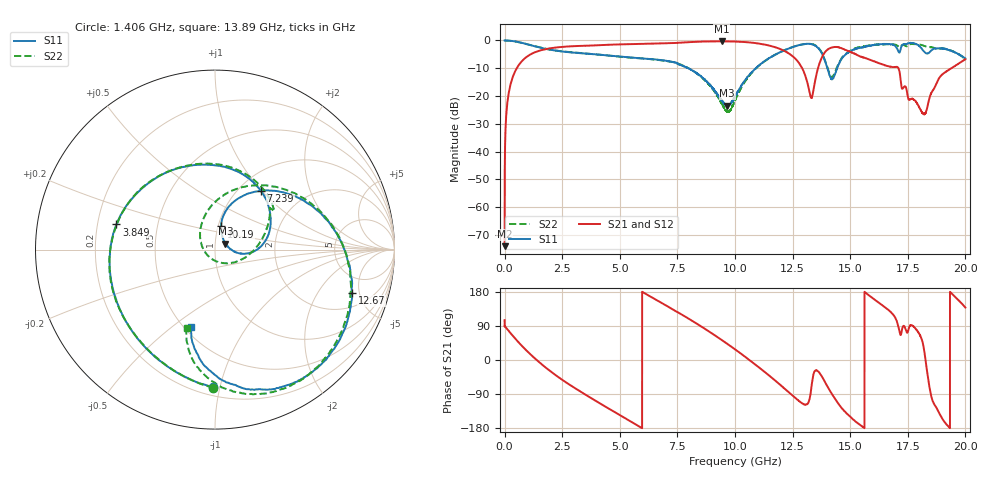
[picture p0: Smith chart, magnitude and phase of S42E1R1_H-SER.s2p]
! Created Wed Nov 25 21:31:11 2020
# khz S ma R 50
! 2 Port Network Data from SP1.SP block
! freq  magS11  angS11  magS21  angS21  magS12  angS12  magS22  angS22
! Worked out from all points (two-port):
!   20001 points, 300 kHz to 20 GHz, reference 50 ohm
!   highest |S21| = -0.32 dB at 9.429 GHz (marker M1); lowest = -74.1 dB at 300 kHz (marker M2)
!   |S21| within 3 dB of the highest: 1.675 GHz to 12.03 GHz (10.35 GHz wide, 151 % of centre); 14.01 GHz to 14.77 GHz (753.6 MHz wide, 5.24 % of centre)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
!   lowest |S11| = -23.5 dB at 9.663 GHz (marker M3), VSWR 1.14, Z = 56 + j3.78 ohm
!   |S11| at or under -10 dB: 7.968565 GHz to 7.970692 GHz (2.127 MHz wide, 0.0267 % of centre); 7.972 GHz to 10.9 GHz (2.929 GHz wide, 31 % of centre); 14.01 GHz to 14.44 GHz (424.7 MHz wide, 2.99 % of centre)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
!   |S22| runs from -25.8 to 0.0 dB; largest |S21 - S12| = 0.012
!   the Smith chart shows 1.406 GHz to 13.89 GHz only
!   S11 on the Smith chart (normalised r, x): 1.406 GHz: 0.26, -0.95; 3.849 GHz: 0.28, +0.12; 7.239 GHz: 1.26, +0.99; 10.19 GHz: 1.03, +0.27; 12.67 GHz: 3.16, -4.21; 13.89 GHz: 0.55, -0.58
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300  0.9984 -0.2  0.0001982 105.2  0.0002223 95.0  0.9986 -0.3
107300  0.9968 -7.9  0.06836 81.9  0.06863 82.0  0.9976 -7.8
255300  0.9847 -18.7  0.1603 71.1  0.1611 71.0  0.9866 -18.6
1406300  0.7677 -90.7  0.6329 -0.7  0.6326 -0.8  0.7705 -90.7
3334300  0.5886 -175.9  0.7988 -84.9  0.7984 -84.9  0.5921 -173.6
3849300  0.5666 165.7  0.8132 -103.9  0.8136 -103.9  0.5659 166.8
6667300  0.4492 71.3  0.8839 155.7  0.8818 155.6  0.4463 61.4
7239300  0.4137 51.6  0.8947 135.7  0.8955 135.6  0.4136 41.4
9429300  0.08355 3.5  0.9641 52.5  0.9639 52.5  0.07229 -74.4
9663300  0.06715 30.0  0.9599 42.7  0.9623 42.7  0.05213 -124.1
1.00003e7  0.09786 68.1  0.9541 28.1  0.9543 28.2  0.08311 157.1
1.01853e7  0.1335 75.3  0.9483 20.0  0.9478 20.0  0.1207 133.6
1.16163e7  0.5182 36.4  0.7827 -47.8  0.7812 -47.8  0.5179 39.9
1.26713e7  0.7998 -17.5  0.4444 -102.8  0.4504 -102.5  0.8014 -19.8
1.33343e7  0.8545 -62.4  0.09385 -63.4  0.09477 -64.3  0.8591 -66.6
1.38923e7  0.4461 -107.1  0.6056 -56.4  0.604 -56.7  0.4584 -109.9
1.42273e7  0.2016 -71.8  0.7513 -91.6  0.7515 -91.5  0.2211 -72.8
1.48823e7  0.5938 -61.0  0.6527 -143.1  0.6531 -143.3  0.6071 -61.0
1.66673e7  0.8602 -140.5  0.3438 131.7  0.336 132.4  0.8568 -138.0
1.81993e7  0.638 161.4  0.04719 29.3  0.04794 29.5  0.7964 159.5
1.89063e7  0.72 151.4  0.2241 -145.3  0.2228 -145.5  0.7132 141.7
2e7  0.4744 115.6  0.4578 138.4  0.4605 139.0  0.4515 109.7
